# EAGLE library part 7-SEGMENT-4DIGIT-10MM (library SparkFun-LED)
4 Digit 7 Segment Display This is a part for the 4-Digit 7-segment LEDs from Young Sun. Different from the Digikey LEDs, all 16 pins are used. The LONGPADS Variant is used for a test jig, but you may like it because there is more pad to solder to. If you are concerned about routing space, the standard works just fine though. Datasheets: Red Yellow Kelly Green Blue White SparkFun Products Raw Components 7-Segment Display - 4-Digit (Red) (COM-09483) 7-Segment Display - 4-Digit (Yellow) (COM-09480) 7-Segment Display - 4-Digit (Kelly Green) (COM-09482) 7-Segment Display - 4-Digit (Blue) (COM-09481) 7-Segment Display - 4-Digit (White) ( COM-10931) Serial Controlled SparkFun 7-Segment Serial Display - Red (COM-11441) SparkFun 7-Segment Serial Display - Yellow (COM-11443) SparkFun 7-Segment Serial Display - Kelly Green (COM-11440) SparkFun 7-Segment Serial Display - Blue (COM-11442) SparkFun 7-Segment Serial Display - White (COM-11629) Other SparkFun BigTime Watch Kit (KIT-11734)
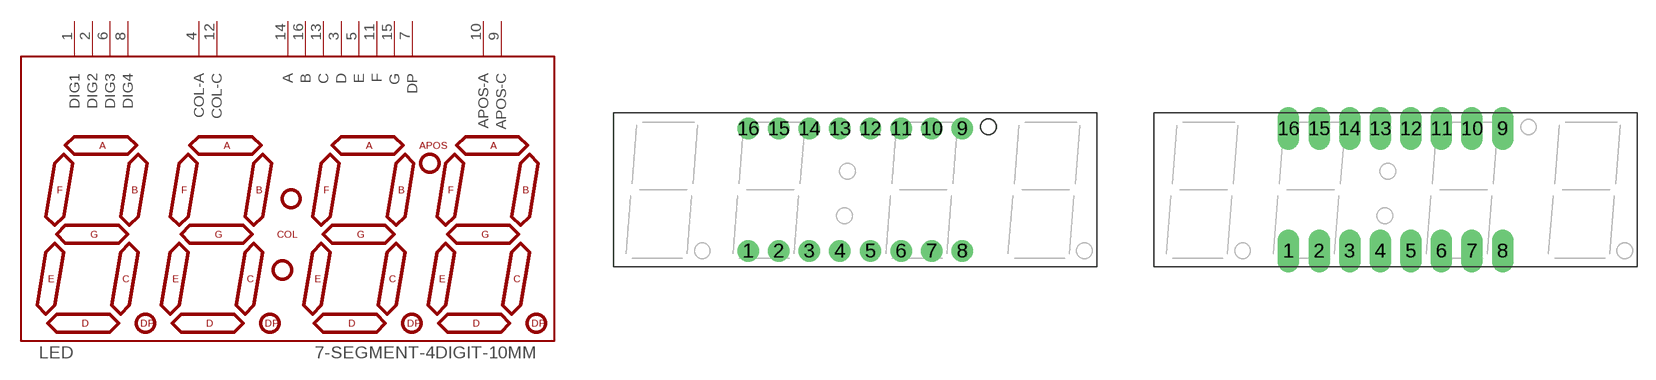
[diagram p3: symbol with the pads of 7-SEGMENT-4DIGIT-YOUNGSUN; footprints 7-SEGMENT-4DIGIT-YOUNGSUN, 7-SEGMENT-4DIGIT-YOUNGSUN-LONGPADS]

Designator prefix LED

## 7-SEGMENT-4DIGIT-10MM-RED (PROD_ID: COMP-09493; VALUE: YSD-439AR6B-35)  [7-SEGMENT-4DIGIT-YOUNGSUN]
1  DIG1
2  DIG2
3  D
4  COL-A
5  E
6  DIG3
7  DP
8  DIG4
9  APOS-C
10  APOS-A
11  F
12  COL-C
13  C
14  A
15  G
16  B

## 7-SEGMENT-4DIGIT-10MMLONGPADS-RED (PROD_ID: COMP-09493; VALUE: YSD-439AR6B-35)  [7-SEGMENT-4DIGIT-YOUNGSUN-LONGPADS]
Pads as for 7-SEGMENT-4DIGIT-YOUNGSUN

## 7-SEGMENT-4DIGIT-10MM-YELLOW (PROD_ID: COMP-09654; VALUE: YSD-439AY2B-35)  [7-SEGMENT-4DIGIT-YOUNGSUN]
Pads as for 7-SEGMENT-4DIGIT-YOUNGSUN

## 7-SEGMENT-4DIGIT-10MM-KGREEN (PROD_ID: COMP-09665; VALUE: YSD-439AK2B-35)  [7-SEGMENT-4DIGIT-YOUNGSUN]
Pads as for 7-SEGMENT-4DIGIT-YOUNGSUN

## 7-SEGMENT-4DIGIT-10MM-BLUE (PROD_ID: COMP-09664; VALUE: YSD-439AB4B-35)  [7-SEGMENT-4DIGIT-YOUNGSUN]
Pads as for 7-SEGMENT-4DIGIT-YOUNGSUN

## 7-SEGMENT-4DIGIT-10MM-WHITE (PROD_ID: COMP-11430; VALUE: WD03942-white / ATA3492BW)  [7-SEGMENT-4DIGIT-YOUNGSUN]
Pads as for 7-SEGMENT-4DIGIT-YOUNGSUN

## Footprint 7-SEGMENT-4DIGIT-YOUNGSUN (pad centres in mm)
This is a package for the 4-digit 7-segment RED LED from Young Sun.
drill 0.8 pad 1.778: 1 -8.89,-5.08; 2 -6.35,-5.08; 3 -3.81,-5.08; 4 -1.27,-5.08; 5 1.27,-5.08; 6 3.81,-5.08; 7 6.35,-5.08; 8 8.89,-5.08; 9 8.89,5.08; 10 6.35,5.08; 11 3.81,5.08; 12 1.27,5.08; 13 -1.27,5.08; 14 -3.81,5.08; 15 -6.35,5.08; 16 -8.89,5.08

## Footprint 7-SEGMENT-4DIGIT-YOUNGSUN-LONGPADS (pad centres in mm)
drill 1.016 pad 1.778 long: 1 -8.89,-5.08; 2 -6.35,-5.08; 3 -3.81,-5.08; 4 -1.27,-5.08; 5 1.27,-5.08; 6 3.81,-5.08; 7 6.35,-5.08; 8 8.89,-5.08; 9 8.89,5.08; 10 6.35,5.08; 11 3.81,5.08; 12 1.27,5.08; 13 -1.27,5.08; 14 -3.81,5.08; 15 -6.35,5.08; 16 -8.89,5.08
